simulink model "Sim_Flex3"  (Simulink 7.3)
settings: Solver=ode4  StartTime=0.0  StopTime=20  RelTol=1e-3
InitFcn:
  | r2d= 180/pi; d2r=1/r2d; Ts=0.04;                  % Radian to degree converts
  | [Afls,Bfls,Cfls,Dfls]= vehicle_flex_s;            % Shuttle Ascent, Max_Q, T=55 sec, Flex Vehicle with Slosh and TWD
  | [Aflz,Bflz,Cflz,Dflz]= vehicle_flex_z;            % Discrete Shuttle Plant Model at Max-Q (Flex Vehicle, Actuators, Sensors)
  | [Alfc,Blfc,Clfc,Dlfc]= lateral_fcs;               % Lateral Flight Control System
  | [Apfc,Bpfc,Cpfc,Dpfc]= pitch_fcs;                 % Pitch Flight Control System
  | [Azpl,Bzpl,Czpl,Dzpl]= vehi_plant_z;              % Load Discrete Plant (Vehi,Actuat,Sensors)
  | [Acts,Bcts,Ccts,Dcts]= actuators_5s;              % System of Five Actuators
  | [Actz,Bctz,Cctz,Dctz]= actuators_5z;              % System of Five Actuators, Z-Transform
  | [Asz, Bsz, Csz, Dsz] = sensors_z;                 % IMU, Gyro, Accelerometer Sensors, Z-transform
  | [Aol, Bol, Col, Dol] = open_loop;                 % Open-Loop System (Plant + FCS)
  | load TVC.Mat -ascii                               % Shuttle Stage-1 TVC Matrix at Max-Q
StopFcn:
  | Pl
undefined symbols (not defined in the file or in its folder): Aol, Bol, Col, Dol

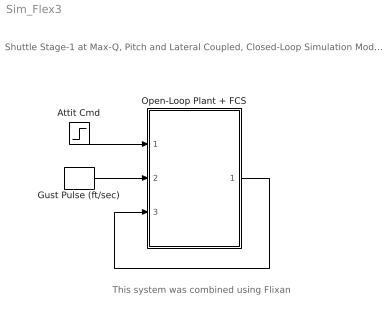
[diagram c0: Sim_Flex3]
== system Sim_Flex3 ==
  note: Shuttle Stage-1 at Max-Q, Pitch and Lateral Coupled, Closed-Loop Simulation Model-3
  note: This system was combined using Flixan
  Attit Cmd : Step  Time=0  After=[1, 0, 0]*d2r
  Gust Pulse (ft/sec) : DiscretePulseGenerator  PulseType=Time based  Amplitude=00  Period=200  PulseWidth=2  PhaseDelay=0.12  SampleTime=1
  Open-Loop Plant + FCS : Subsystem
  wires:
  Open-Loop Plant + FCS/1(TVCo) -> Open-Loop Plant + FCS/3(TVC)
  Gust Pulse (ft/sec)/1 -> Open-Loop Plant + FCS/2(WG)
  Attit Cmd/1 -> Open-Loop Plant + FCS/1(attc)

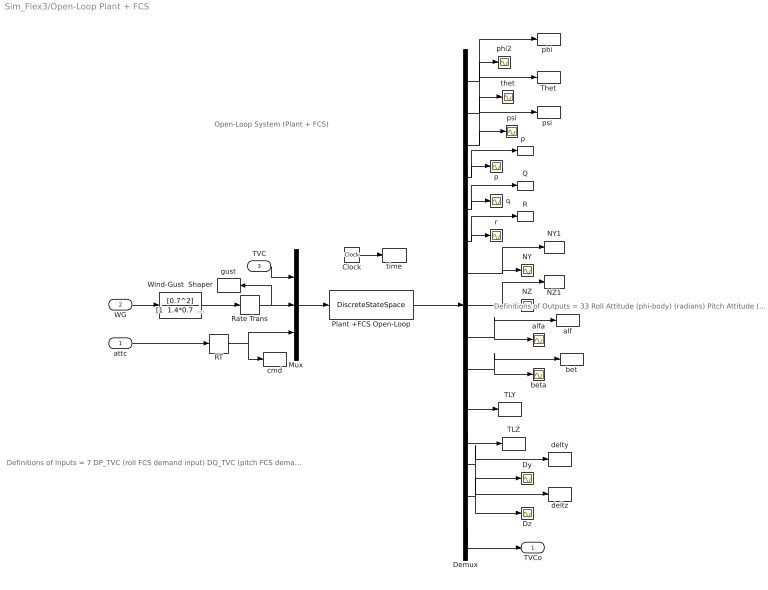
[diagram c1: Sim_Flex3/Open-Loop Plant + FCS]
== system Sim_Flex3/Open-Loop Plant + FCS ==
  note: Definitions of Outputs = 33 Roll Attitude (phi-body) (radians) Pitch Attitude (thet-bdy) (radians) Yaw Attitude (psi-body) (radians) Roll Rate Gyro (p-flex) (rad/sec) Pitch Rate Gyro (q-flex) (rad/sec) Yaw Rate Gyro (r-flex) (rad/sec) Accelerom # 1, Y-ddot Accelerat. (ft/sec^2) Accelerom # 2, Z-ddot Accelerat. (ft/sec^2) Angle of attack, alfa, (radians) Angle of sideslip, beta, (radian) Load-Torque Pitch TLY-Eng-1 Load-Torque Pitch TLY-Eng-2 Load-Torque Pitch TLY-Eng-3 Load-Torque Pitch TLY-Eng-4 Load-Torque Pitch TLY-Eng-5 Load-Torque Yaw TLZ-Eng-1 Load-Torque Yaw TLZ-Eng-2 Load-Torque Yaw TLZ-Eng-3 Load-Torque Yaw TLZ-Eng-4 Load-Torque Yaw TLZ-Eng-5 Engine # 1 Pitch Deflection dy-1 (rad) Engine # 2 Pitch Deflection dy-2 (rad) Engine # 3 Pitch Deflection dy-3 (rad) Engine # 4 Pitch Deflection dy-4 (rad) Engine # 5 Pitch Deflection dy-5 (rad) Engine # 1 Yaw Deflection dz-1 (rad) Engine # 2 Yaw Deflection dz-2 (rad) Engine # 3 Yaw Deflection dz-3 (rad) Engine # 4 Yaw Deflection dz-4 (rad) Engine # 5 Yaw Deflection dz-5 (rad) DP_TVC (roll FCS demand output) DQ_TVC (pitch FCS demand output) DR_TVC (yaw FCS demand output)
  note: Definitions of Inputs = 7 DP_TVC (roll FCS demand input) DQ_TVC (pitch FCS demand input) DR_TVC (yaw FCS demand input) Wind Gust Velocity (ft/sec) Theta Attitude Command (rad) Phi Attitude Command (rad) Psi Attitude Command (rad)
  note: Open-Loop System (Plant + FCS)
  attc : Inport  PortDimensions=3  OutDataType=sfix(16)  OutScaling=2^0
  WG : Inport  Port=2  PortDimensions=1  OutDataType=sfix(16)  OutScaling=2^0
  TVC : Inport  Port=3  PortDimensions=3  OutDataType=sfix(16)  OutScaling=2^0
  Clock : Clock
  Demux : Demux  Outputs=[1,1,1,1,1,1,1,1,1,1, 5,5, 5,5, 3]
  Dy : Scope
  Dz : Scope
  Mux : Mux  Inputs=[3, 1, 3]
  NY : Scope
  NY1 : ToWorkspace  VariableName=Ny  SampleTime=-1  SaveFormat=Array
  NZ : Scope
  NZ1 : ToWorkspace  VariableName=Nz  SampleTime=-1  SaveFormat=Array
  Plant +FCS Open-Loop : DiscreteStateSpace  A=Aol  B=Bol  C=Col  D=Dol  SampleTime=Ts
  Q : ToWorkspace  VariableName=q  SampleTime=-1  SaveFormat=Array
  R : ToWorkspace  VariableName=r  SampleTime=-1  SaveFormat=Array
  RT : RateTransition
  Rate Trans : RateTransition
  TLY : ToWorkspace  VariableName=TLy  SampleTime=-1  SaveFormat=Array
  TLZ : ToWorkspace  VariableName=TLz  SampleTime=-1  SaveFormat=Array
  Thet : ToWorkspace  VariableName=theta  SampleTime=-1  SaveFormat=Array
  Wind-Gust  Shaper : TransferFcn  Numerator=[0.7^2]  Denominator="[1  1.4*0.7  0.7^2]"
  alf : ToWorkspace  VariableName=alpha  SampleTime=-1  SaveFormat=Array
  alfa : Scope
  bet : ToWorkspace  VariableName=beta  SampleTime=-1  SaveFormat=Array
  beta : Scope
  cmd : ToWorkspace  VariableName=cmd  SampleTime=-1  SaveFormat=Array
  delty : ToWorkspace  VariableName=delty  SampleTime=-1  SaveFormat=Array
  deltz : ToWorkspace  VariableName=deltz  SampleTime=-1  SaveFormat=Array
  gust : ToWorkspace  VariableName=Gust  SampleTime=-1  SaveFormat=Array
  p : Scope
  "p  " : ToWorkspace  VariableName=p  SampleTime=-1  SaveFormat=Array
  "phi " : ToWorkspace  VariableName=phi  SampleTime=-1  SaveFormat=Array
  phi2 : Scope
  psi : Scope
  "psi " : ToWorkspace  VariableName=psi  SampleTime=-1  SaveFormat=Array
  q : Scope
  r : Scope
  thet : Scope
  time : ToWorkspace  VariableName=time  SampleTime=-1  SaveFormat=Array
  TVCo : Outport  OutDataType=sfix(16)  OutScaling=2^0
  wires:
  Demux/7 -> NY/1, NY1/1
  Demux/8 -> NZ/1, NZ1/1
  Demux/9 -> alfa/1, alf/1
  Demux/10 -> beta/1, bet/1
  Demux/1 -> phi2/1, "phi "/1
  Demux/2 -> thet/1, Thet/1
  Demux/3 -> psi/1, "psi "/1
  Demux/4 -> p/1, "p  "/1
  Demux/5 -> q/1, Q/1
  Demux/6 -> r/1, R/1
  Demux/14 -> Dz/1, deltz/1
  Demux/13 -> Dy/1, delty/1
  WG/1 -> Wind-Gust  Shaper/1
  attc/1 -> RT/1
  Rate Trans/1 -> Mux/2, gust/1
  Mux/1 -> Plant +FCS Open-Loop/1
  TVC/1 -> Mux/1
  Plant +FCS Open-Loop/1 -> Demux/1
  Demux/15 -> TVCo/1
  Clock/1 -> time/1
  Demux/11 -> TLY/1
  Demux/12 -> TLZ/1
  RT/1 -> Mux/3, cmd/1
  Wind-Gust  Shaper/1 -> Rate Trans/1
